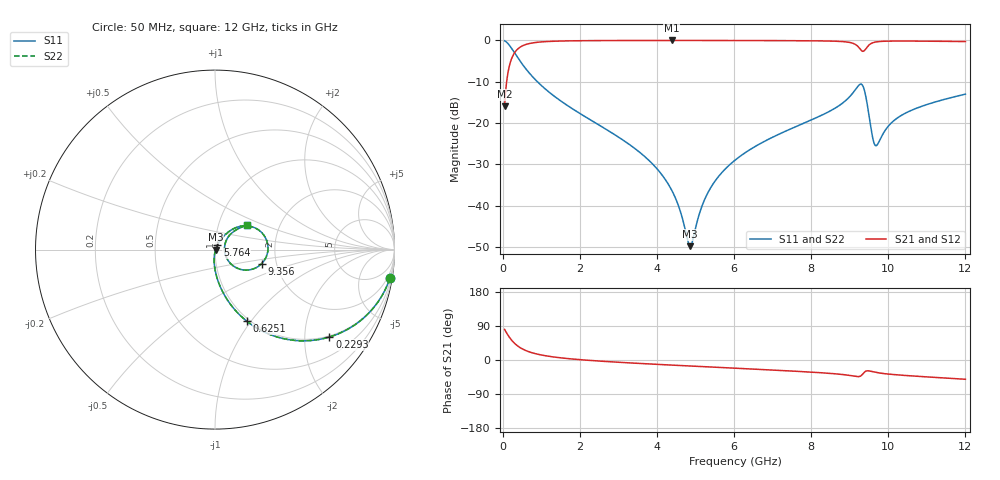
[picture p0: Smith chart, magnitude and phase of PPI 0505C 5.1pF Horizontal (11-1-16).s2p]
# MHz S MA R 50
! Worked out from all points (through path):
!   1601 points, 50 MHz to 12 GHz, reference 50 ohm
!   highest |S21| = -0.03 dB at 4.382 GHz (marker M1); lowest = -15.9 dB at 50 MHz (marker M2)
!   group delay of S21, straight-line fit = 17 ps
!   lowest |S11| = -49.8 dB at 4.86 GHz (marker M3), VSWR 1.01, Z = 50.3 - j0.1 ohm
!   |S11| at or under -10 dB: 898.6 MHz to end of sweep
!   |S22| runs from -49.8 to -0.1 dB; largest |S21 - S12| = 0
!   S11 on the Smith chart (normalised r, x): 50 MHz: 1, -12; 229.2 MHz: 0.97, -2.64; 625.1 MHz: 0.97, -0.96; 5.764 GHz: 1.02, +0.05; 9.356 GHz: 1.67, -0.28; 12 GHz: 1.37, +0.39
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50  0.9871 -9.4  0.1599 80.6  0.1599 80.6  0.9871 -9.4
147.0938  0.9025 -26.0  0.4303 64.0  0.4303 64.0  0.9025 -26.0
229.25  0.8021 -37.4  0.5966 52.6  0.5966 52.6  0.8021 -37.4
408.5  0.6003 -54.4  0.7989 35.6  0.7989 35.6  0.6003 -54.4
625.0938  0.4375 -66.0  0.8981 23.9  0.8981 23.9  0.4375 -66.0
1103.094  0.2583 -78.3  0.9645 11.3  0.9645 11.3  0.2583 -78.3
2044.156  0.1268 -88.5  0.9898 0.6  0.9898 0.6  0.1268 -88.5
3336.25  0.05286 -95.1  0.9958 -7.9  0.9958 -7.9  0.05286 -95.1
4038.312  0.02671 -95.5  0.9965 -11.7  0.9965 -11.7  0.02671 -95.5
4381.875  0.01544 -92.1  0.9966 -13.4  0.9966 -13.4  0.01544 -92.1
4859.875  0.003237 -17.9  0.9965 -15.8  0.9965 -15.8  0.003237 -17.9
5270.656  0.01284 56.7  0.9962 -17.9  0.9962 -17.9  0.01284 56.7
5763.594  0.02752 62.0  0.9956 -20.3  0.9956 -20.3  0.02752 62.0
6025  0.03549 62.2  0.9952 -21.6  0.9952 -21.6  0.03549 62.2
8019.156  0.1097 54.5  0.987 -32.2  0.987 -32.2  0.1097 54.5
9094.656  0.2349 33.6  0.9163 -42.4  0.9163 -42.4  0.2349 33.6
9356.062  0.2709 -16.9  0.7381 -34.8  0.7381 -34.8  0.2709 -16.9
9505.438  0.1193 -42.0  0.8829 -28.9  0.8829 -28.9  0.1193 -42.0
9654.812  0.05401 -7.2  0.9502 -32.2  0.9502 -32.2  0.05401 -7.2
10013.31  0.09298 42.3  0.9783 -37.2  0.9783 -37.2  0.09298 42.3
10670.56  0.147 44.0  0.9792 -42.4  0.9792 -42.4  0.147 44.0
12000  0.2235 37.1  0.966 -50.9  0.966 -50.9  0.2235 37.1
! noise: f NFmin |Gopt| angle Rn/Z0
50  0.0005284  0.9079  1.998  0.00126
1372  0.004872  0.7256  5.135  0.00352
2701  0.008018  0.6808  9.218  0.00483
4031  0.0109  0.6561  13.32  0.005966
5360  0.01378  0.6432  17.37  0.007146
6682  0.017  0.6424  21.34  0.008696
8012  0.02275  0.676  25.34  0.01292
9341  0.1754  0.9437  29.93  0.6508
1.067e+04  0.03128  0.6901  33.38  0.01808
1.2e+04  0.03091  0.6587  36.77  0.01565
